TYPE Nci_SingleEntry :
STRUCT
        SyncVelo                       :REAL; //给进速度
		SyncAcc                        :REAL; //给进加速度
		fx ,fy,fz                      :REAL; //插补轴目标位置
        fQ1,fQ2,fQ3,fQ4,fQ5            :REAL; //辅助轴目标位置
		
        fCenterX,fCenterY,fCenterZ     :REAL; //圆弧插补圆心位置
		bClockwise                     :BOOL; //顺、逆时针方向
		iPlane                         :UDINT;//插补形式
END_STRUCT
END_TYPE
